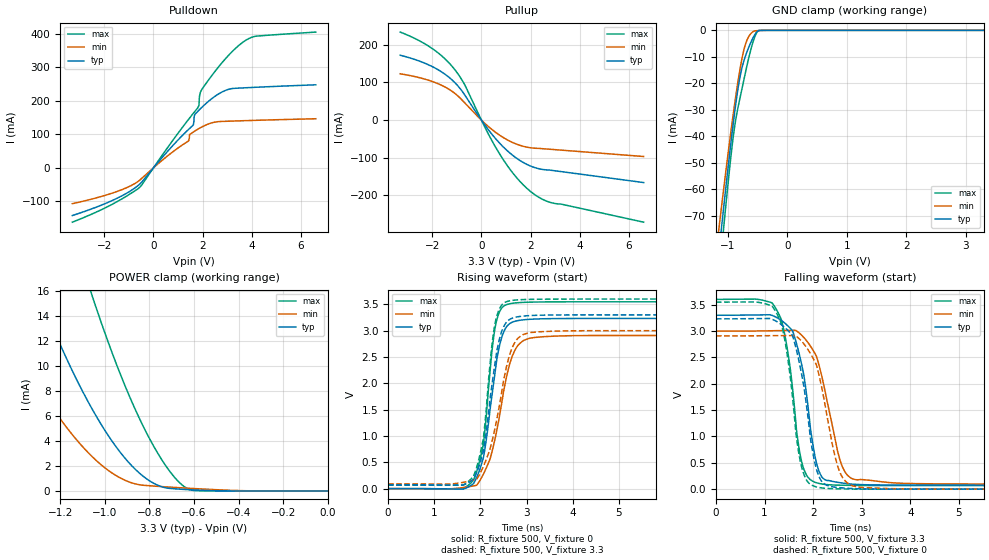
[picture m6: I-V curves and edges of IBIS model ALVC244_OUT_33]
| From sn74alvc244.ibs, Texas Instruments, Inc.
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[Model]   ALVC244_OUT_33
Model_type  3-state
Enable   Active-Low
Vref =   0
Rref =   500
Cref =   50p
Vmeas =   1.5
| variable   typ   min   max
C_comp   6.04pF   5.27pF   7.08pF
| C_pullup   8.39pF   6.15pF   9.77pF
| C_pulldown   7.96pF   1.77pF   20.27pF
| C_tri-state   6.04pF   5.27pF   7.08pF
[Temperature Range]   40   100   -40
| Ambient temperature   25   85   -40
[Voltage range]   3.3   3   3.6
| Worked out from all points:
|   slope of the pulldown table from 0 to 0.495 V, typ, clamps not added: 11.6 ohm
|   slope of the pullup table from 0 to 0.495 V, typ, clamps not added: 11.5 ohm
|   GND clamp passes 1 mA (typ) near -0.53 V on its own axis
|   POWER clamp passes 1 mA (typ) near -0.82 V on its own axis
|   rising waveform, R_fixture 500, V_fixture 0: 20-80 % time 306ps typ, 407ps min, 249ps max; typ from 0 V to 3.23 V
|   falling waveform, R_fixture 500, V_fixture 3.3: 20-80 % time 330ps typ, 416ps min, 287ps max; typ from 3.3 V to 0.073 V
|   rising waveform, R_fixture 500, V_fixture 3.3: 20-80 % time 301ps typ, 418ps min, 252ps max; typ from 0.073 V to 3.3 V
|   falling waveform, R_fixture 500, V_fixture 0: 20-80 % time 332ps typ, 385ps min, 285ps max; typ from 3.23 V to 0 V
[GND Clamp]
| ALVC244_OUT_33
|   Voltage   I(typ)   I(min)   I(max)
-3.3V     -594.4mA   -529.6mA   -658.2mA
-1.16V    -85.69mA   -76.57mA   -95.55mA
-1.135V   -80.34mA   -71.83mA   -89.56mA
-1.11V    -75.03mA   -67.13mA   -83.61mA
-1.065V   -65.61mA   -58.78mA   -73.07mA
-920mV    -36.97mA   -33.27mA   -41.98mA
-870mV    -28.2mA    -25.22mA   -33.97mA
-805mV    -18.64mA   -15.77mA   -26.42mA
-690mV    -8.749mA   -4.308mA   -14.39mA
-560mV    -2.112mA   -312.7uA   -3.216mA
-475mV    -33.84uA   -89.41uA   -29.91uA
3.3V      139.2pA    2.263uA    18.29pA
[POWER Clamp]
| ALVC244_OUT_33
|   Voltage   I(typ)   I(min)   I(max)
-3.3V     153.6mA    107.4mA    219.7mA
-1.515V   26.5mA     15.47mA    46.12mA
-1.39V    20.13mA    11.19mA    36.8mA
-1.295V   15.71mA    8.296mA    30.16mA
-1.175V   10.71mA    5.163mA    22.42mA
-1.055V   6.486mA    2.711mA    15.5mA
-950mV    3.54mA     1.231mA    10.22mA
-845mV    1.423mA    493.2uA    5.796mA
-745mV    332.8uA    345.7uA    2.502mA
-655mV    131.2uA    246.7uA    499.2uA
-600mV    76.89uA    190.3uA    26.37uA
-48.03fV  139.2pA    584pA      20.85pA
[Pulldown]
| ALVC244_OUT_33
|   Voltage   I(typ)   I(min)   I(max)
-3.3V     -142.2mA   -106.8mA   -162mA
-520mV    -45.93mA   -34.15mA   -55.1mA
1.615V    126.9mA    106.4mA    162mA
1.665V    155.6mA    108.8mA    166.5mA
1.81V     168.9mA    115.4mA    179.2mA
1.85V     171.8mA    117.1mA    184.6mA
1.885V    174.4mA    118.6mA    218.4mA
2.005V    182.9mA    123.2mA    237.8mA
2.8V      226.5mA    138.3mA    314.4mA
3.56V     238mA      140.2mA    370.1mA
4.16V     240.1mA    141.6mA    392.3mA
6.6V      247.5mA    146.3mA    404.6mA
[Pullup]
| ALVC244_OUT_33
|   Voltage   I(typ)   I(min)   I(max)
-3.3V     172.1mA    122.8mA    233.6mA
-2.04V    143.3mA    103.3mA    191.7mA
-1.55V    124.9mA    90.03mA    166.7mA
-1.135V   102.9mA    73.49mA    138.3mA
-685mV    67.23mA    46.15mA    94.4mA
200mV     -18.44mA   -12.39mA   -26.59mA
785mV     -64.42mA   -42.2mA    -94.61mA
1.415V    -100.8mA   -63.67mA   -151.7mA
2.045V    -123.5mA   -74.13mA   -192.2mA
2.445V    -130.9mA   -75.97mA   -209.3mA
2.85V     -133.6mA   -78.01mA   -219.7mA
6.6V      -166.2mA   -96.97mA   -271.5mA
[Ramp]
| ALVC244_OUT_33
| variable   typ   min   max
dV/dt_r   1.95/3.19E-10   1.75/4.10E-10   2.13/2.62E-10
dV/dt_f   1.94/3.49E-10   1.76/4.25E-10   2.12/3.08E-10
R_load = 500
[Rising Waveform]
| ALVC244_OUT_33
R_fixture =   500
C_fixture =   0
L_fixture =   0
V_fixture =   0
V_fixture_min = 0
V_fixture_max = 0
|   Time   V(typ)   V(min)   V(max)
0s        72.42pV    3.267nV    61.17pV
1.63ns    -10.17mV   20.3mV     1.264mV
1.845ns   90.14mV    51.12mV    153.3mV
2.065ns   589.7mV    276.5mV    843.7mV
2.24ns    1.701V     663mV      2.526V
2.35ns    2.42V      1.084V     3.188V
2.535ns   3.03V      1.989V     3.483V
2.82ns    3.192V     2.727V     3.531V
4.32ns    3.232V     2.907V     3.548V
50ns      3.232V     2.909V     3.548V
[Falling Waveform]
| ALVC244_OUT_33
R_fixture =   500
C_fixture =   0
L_fixture =   0
V_fixture =   3.3
V_fixture_min = 3
V_fixture_max = 3.6
|   Time   V(typ)   V(min)   V(max)
0s        3.3V       3V         3.6V
1.155ns   3.297V     3.006V     3.532V
1.37ns    3.185V     3.01V      3.125V
1.575ns   3.006V     3.014V     1.916V
1.805ns   2.178V     2.881V     386.1mV
2.055ns   547.5mV    2.543V     125.5mV
2.305ns   164.6mV    1.589V     84.99mV
2.705ns   104mV      265.4mV    73.08mV
3.88ns    77.45mV    109.6mV    68.22mV
50ns      72.85mV    89.69mV    66.09mV
[Rising Waveform]
| ALVC244_OUT_33
R_fixture =   500
C_fixture =   0
L_fixture =   0
V_fixture =   3.3
V_fixture_min = 3
V_fixture_max = 3.6
|   Time   V(typ)   V(min)   V(max)
0s        72.85mV    89.69mV    66.09mV
1.63ns    66.57mV    119.7mV    69.65mV
1.845ns   174.2mV    160.4mV    226mV
2.065ns   719.8mV    423.2mV    959.8mV
2.24ns    1.907V     859mV      2.648V
2.34ns    2.519V     1.249V     3.229V
2.515ns   3.094V     2.111V     3.529V
2.78ns    3.258V     2.822V     3.583V
4.315ns   3.3V       2.999V     3.6V
50ns      3.3V       3V         3.6V
[Falling Waveform]
| ALVC244_OUT_33
R_fixture =   500
C_fixture =   0
L_fixture =   0
V_fixture =   0
V_fixture_min = 0
V_fixture_max = 0
|   Time   V(typ)   V(min)   V(max)
0s        3.232V     2.909V     3.548V
1.155ns   3.224V     2.913V     3.472V
1.365ns   3.108V     2.914V     3.067V
1.575ns   2.914V     2.914V     1.743V
1.815ns   1.905V     2.749V     268.4mV
2.035ns   497mV      2.417V     50.71mV
2.265ns   79.58mV    1.492V     15.32mV
2.62ns    23.11mV    200.7mV    4.662mV
3.51ns    828.5uV    12.17mV    560.8uV
50ns      374.7nV    753.3nV    235.2nV
